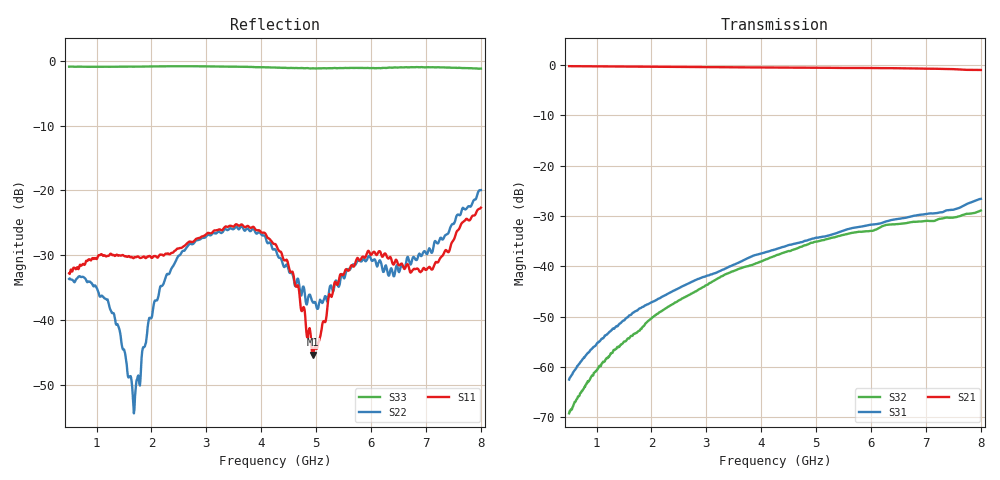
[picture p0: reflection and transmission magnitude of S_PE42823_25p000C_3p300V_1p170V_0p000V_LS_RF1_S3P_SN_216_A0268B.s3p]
! Device ID: PE42823
! File Path: z:\PE42823\DSPLOTS2\25p000C\3p300\LS_RF1\PE42823_25p000C_3p300V_1p170V_0p000V_LS_RF1_S3P_SN_216_A0268B.s3p
! Serial: 216
! Lot: A0268B
! Temp: 25.000C
! VDD: 3.300
! VSS: 0.000
! Control_Hi: 1.170
! Control_Lo: 0.000
! Logic State: LS_RF1
! Port 1: RFC
! Port 2: RF1
! Port 3: RF2
! ThroughPath:1-2
! IDD: 0.000121413685
! ISS/IDD2: -3.24892458e-009
! IDMM3/IDD3: 0
! Comment:
#  Hz  S  RI  R  50
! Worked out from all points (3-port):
!   751 points, 500 MHz to 8 GHz, reference 50 ohm
!   strongest paths, dB at 500 MHz, 2.37 GHz, 4.25 GHz, 6.13 GHz, 8 GHz:
!     S21: -0.2, -0.4, -0.5, -0.6, -1.0
!     S31: -62.5, -45.1, -36.6, -31.6, -26.6
!     S32: -69.2, -47.6, -37.9, -32.5, -28.9
!   lowest |S11| = -45.4 dB at 4.94 GHz (marker M1), VSWR 1.01, Z = 50.1 + j0.524 ohm
!   |S11| at or under -10 dB: start of sweep to end of sweep
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5e8  0.0229 -0.00131  0.9674 -0.1169  -0.000132 0.000736
     0.968 -0.1165  0.0207 -0.000374  -0.000272 -0.000219
     -0.000128 0.000739  -0.000279 -0.000205  -0.8898 0.1453
1.19e9  0.0292 -0.011  0.9326 -0.2684  -0.000595 0.00201
        0.9322 -0.2696  0.0138 -0.00405  -0.00123 -0.000146
        -0.000595 0.00201  -0.00123 -0.000147  -0.8375 0.33
1.68e9  0.0281 -0.0106  0.8917 -0.3706  -0.00106 0.00331
        0.8914 -0.372  0.00164 0.00095  -0.00214 0.000234
        -0.00106 0.00333  -0.00212 0.000245  -0.7794 0.4536
2.06e9  0.0306 -0.00549  0.8528 -0.4465  -0.00126 0.00436
        0.8522 -0.446  -0.0036 0.0136  -0.00315 0.000769
        -0.00128 0.00437  -0.00315 0.000757  -0.7238 0.545
2.67e9  0.038 0.0111  0.7783 -0.5565  -0.00175 0.00653
        0.7778 -0.5571  0.00131 0.0375  -0.00459 0.0024
        -0.00174 0.00652  -0.00456 0.00241  -0.6164 0.6685
4.25e9  0.0344 0.0174  0.5245 -0.7876  -0.000954 0.0147
        0.5233 -0.7878  0.0296 0.0188  -0.00688 0.0108
        -0.000939 0.0147  -0.00681 0.0107  -0.2567 0.8493
4.94e9  0.0013 0.00522  0.3878 -0.8578  0.00105 0.0188
        0.3878 -0.8578  0.00942 -0.00986  -0.00583 0.0163
        0.00104 0.0188  -0.00581 0.0162  -0.0538 0.8737
5.75e9  -0.0299 -0.00372  0.2149 -0.9106  0.0047 0.024
        0.2129 -0.9118  -0.0263 -0.0113  -0.00138 0.0218
        0.00481 0.0241  -0.00123 0.0219  0.156 0.8674
7.11e9  -0.018 0.0165  -0.1051 -0.9138  0.0131 0.0308
        -0.1066 -0.9137  -0.019 0.027  0.00718 0.0273
        0.0132 0.0309  0.00725 0.0272  0.4519 0.77
8e9  -0.0413 0.0608  -0.3094 -0.8388  0.0182 0.0431
     -0.3095 -0.8386  -0.0612 0.0797  0.00841 0.0349
     0.0183 0.0432  0.00845 0.0349  0.582 0.648
